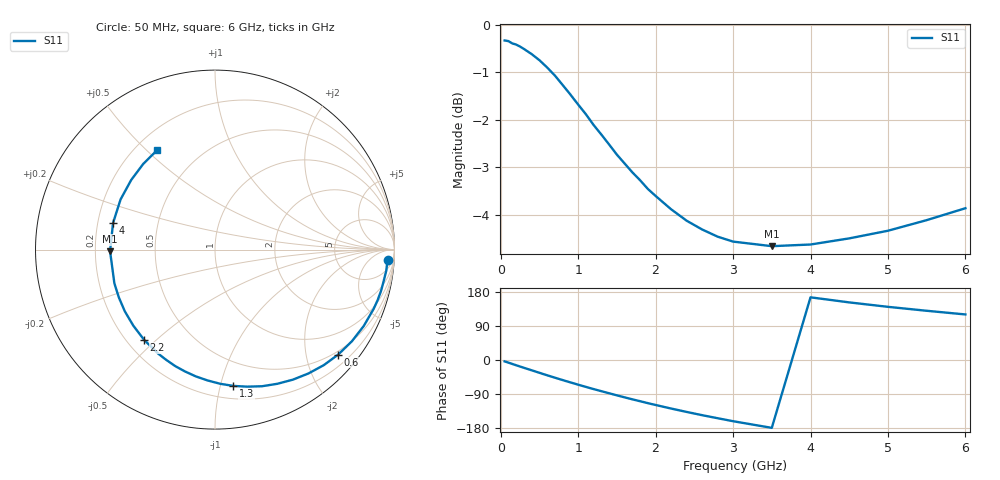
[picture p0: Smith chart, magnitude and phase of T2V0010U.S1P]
! SIEMENS Discrete & RF Semiconductors
! BAS70-04W
! Si Schottky Diode in SOT323
! IF = 0.01 mA
! S-Parameters:  November  1997
# GHz  S  MA  R  50
!  f  S11
! GHz  MAG  ANG
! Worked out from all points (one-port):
!   34 points, 50 MHz to 6 GHz, reference 50 ohm
!   lowest |S11| = -4.7 dB at 3.5 GHz (marker M1), VSWR 3.82, Z = 13.1 - j0.366 ohm
!   |S11| at or under -10 dB: nowhere
!   S11 on the Smith chart (normalised r, x): 50 MHz: 14, -23; 600 MHz: 0.42, -2.66; 1.3 GHz: 0.30, -1.10; 2.2 GHz: 0.27, -0.46; 4 GHz: 0.26, +0.12; 6 GHz: 0.29, +0.54
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0.05  0.9631 -3.6
0.1  0.9615 -7.0
0.2  0.9534 -13.9
0.3  0.9434 -20.6
0.4  0.9316 -27.2
0.5  0.918 -33.8
0.6  0.9018 -40.4
0.7  0.8843 -46.7
0.8  0.8643 -53.0
0.9  0.8445 -59.1
1  0.8243 -65.1
1.1  0.8052 -71.0
1.3  0.7664 -82.3
1.4  0.7481 -87.8
1.6  0.7145 -98.6
1.7  0.6993 -103.8
1.9  0.6717 -113.9
2.2  0.6394 -128.1
2.4  0.622 -137.0
2.6  0.6089 -145.6
2.8  0.5984 -153.6
3  0.5912 -161.5
3.5  0.5847 -179.1
4  0.587 165.4
4.5  0.5958 152.0
5  0.607 140.3
5.5  0.6228 129.9
6  0.641 120.2
